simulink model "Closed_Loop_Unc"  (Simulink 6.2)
settings: Solver=ode23s  StartTime=0.0  StopTime=60  FixedStep=0.04  RelTol=1e-3
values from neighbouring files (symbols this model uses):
  Npv = 45    [run.m]
  r2d = 180/pi    (= 57.2957795131)    [run.m]    (also in Pl.m; pl.m; start.m)
undefined symbols (not defined in the file or in its folder): Ac, As, At, Au, Bc, Bs, Bt, Bu, Cc, Cs, Ct, Cu, Dc, Ds, Dt, Du

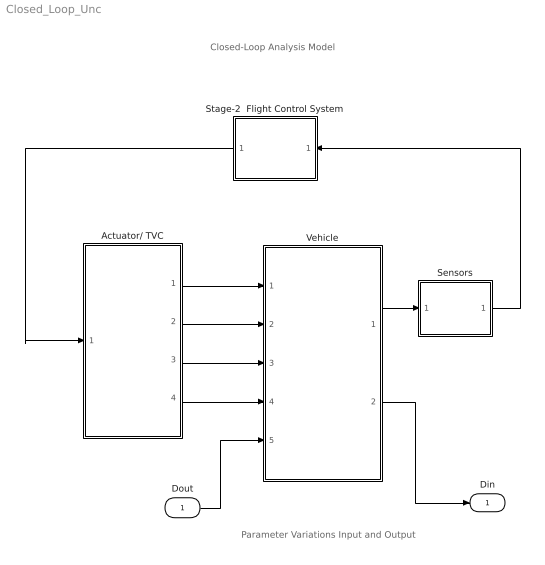
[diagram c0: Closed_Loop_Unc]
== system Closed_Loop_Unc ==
  note: Closed-Loop Analysis Model
  note: Parameter Variations Input and Output
  Dout : Inport  Port=1  LatchInput=off
  Actuator/ TVC : Subsystem
  Sensors : Subsystem
  Stage-2  Flight Control System : Subsystem  Orientation=left
  Vehicle : Subsystem
  Din : Outport
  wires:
  Vehicle/1(meas) -> Sensors/1(meas)
  Actuator/ TVC/1(DY) -> Vehicle/1(DY)
  Actuator/ TVC/2(DY-dd) -> Vehicle/2(DY_dd)
  Actuator/ TVC/3(DZ) -> Vehicle/3(DZ)
  Actuator/ TVC/4(DZ-dd) -> Vehicle/4(DZ_dd)
  Sensors/1(sens) -> Stage-2  Flight Control System/1(sens)
  Stage-2  Flight Control System/1(TVC) -> Actuator/ TVC/1(TVC)
  Vehicle/2(Din) -> Din/1
  Dout/1 -> Vehicle/5(Dout)

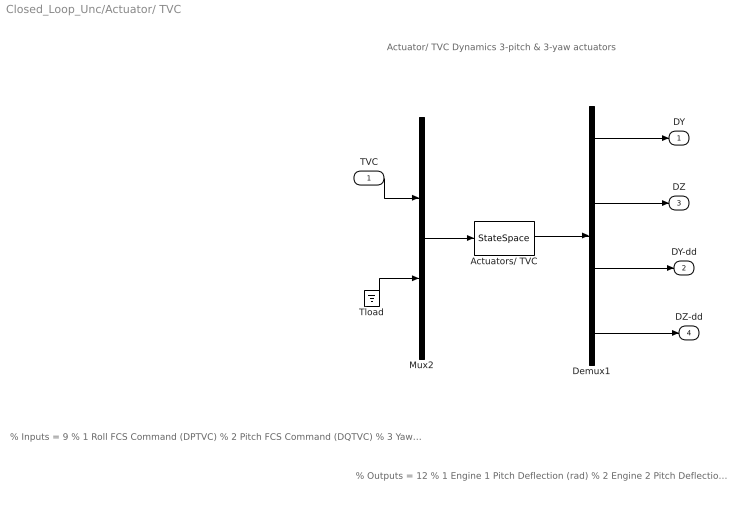
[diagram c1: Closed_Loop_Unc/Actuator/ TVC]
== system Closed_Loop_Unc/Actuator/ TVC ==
  note: % Outputs = 12 % 1 Engine 1 Pitch Deflection (rad) % 2 Engine 2 Pitch Deflection (rad) % 3 Engine 3 Pitch Deflection (rad) % 4 Engine 1 Yaw Deflection (rad) % 5 Engine 2 Yaw Deflection (rad) % 6 Engine 3 Yaw Deflection (rad) % 7 Engine 1 Pitch Accelerat (rad/sec^2) % 8 Engine 2 Pitch Accelerat (rad/sec^2) % 9 Engine 3 Pitch Accelerat (rad/sec^2) % 10 Engine 1 Yaw Accelerat (rad/sec^2) % 11 Engine 2 Yaw Accelerat (rad/sec^2) % 12 Engine 3 Yaw Accelerat (rad/sec^2)
  note: % Inputs = 9 % 1 Roll FCS Command (DPTVC) % 2 Pitch FCS Command (DQTVC) % 3 Yaw FCS Command (DRTVC) % 4 Engine 1 Pitch Load-Torque TLY1 % 5 Engine 2 Pitch Load-Torque TLY2 % 6 Engine 3 Pitch Load-Torque TLY3 % 7 Engine 1 Yaw Load-Torque TLZ1 % 8 Engine 2 Yaw Load-Torque TLZ2 % 9 Engine 3 Yaw Load-Torque TLZ3
  note: Actuator/ TVC Dynamics 3-pitch & 3-yaw actuators
  TVC : Inport  Port=1  LatchInput=off
  Actuators/ TVC : StateSpace  A=At  B=Bt  C=Ct  D=Dt
  Demux1 : Demux  Outputs=[3, 3, 3, 3]
  Mux2 : Mux  Inputs="[3,  6]"
  Tload : Ground
  DY : Outport
  DY-dd : Outport  Port=2
  DZ : Outport  Port=3
  DZ-dd : Outport  Port=4
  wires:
  Demux1/3 -> DY-dd/1
  Demux1/4 -> DZ-dd/1
  Demux1/2 -> DZ/1
  Demux1/1 -> DY/1
  TVC/1 -> Mux2/1
  Tload/1 -> Mux2/2
  Actuators/ TVC/1 -> Demux1/1
  Mux2/1 -> Actuators/ TVC/1

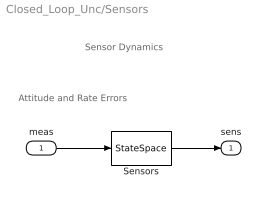
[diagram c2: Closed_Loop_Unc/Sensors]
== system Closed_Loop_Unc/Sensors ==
  note: Attitude and Rate Errors
  note: Sensor Dynamics
  meas : Inport  Port=1  LatchInput=off
  Sensors : StateSpace  A=As  B=Bs  C=Cs  D=Ds
  sens : Outport
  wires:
  Sensors/1 -> sens/1
  meas/1 -> Sensors/1

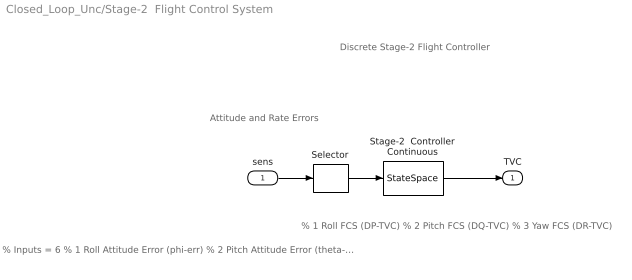
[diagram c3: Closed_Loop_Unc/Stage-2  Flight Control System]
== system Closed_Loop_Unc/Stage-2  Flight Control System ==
  note: Discrete Stage-2 Flight Controller
  note: Attitude and Rate Errors
  note: % Inputs = 6 % 1 Roll Attitude Error (phi-err) % 2 Pitch Attitude Error (theta-err) % 3 Yaw Attitude Error (psi-err) % 4 Roll Rate Error (p-err) % 5 Pitch Rate Error (q-err) % 6 Yaw Rate Error (r-err)
  note: % 1 Roll FCS (DP-TVC) % 2 Pitch FCS (DQ-TVC) % 3 Yaw FCS (DR-TVC)
  sens : Inport  Port=1  LatchInput=off
  Selector : Selector  Elements=[1 3 5 2 4 6]  InputPortWidth=6
  Stage-2  Controller Continuous : StateSpace  A=Ac  B=Bc  C=Cc  D=Dc
  TVC : Outport
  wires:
  sens/1 -> Selector/1
  Stage-2  Controller Continuous/1 -> TVC/1
  Selector/1 -> Stage-2  Controller Continuous/1

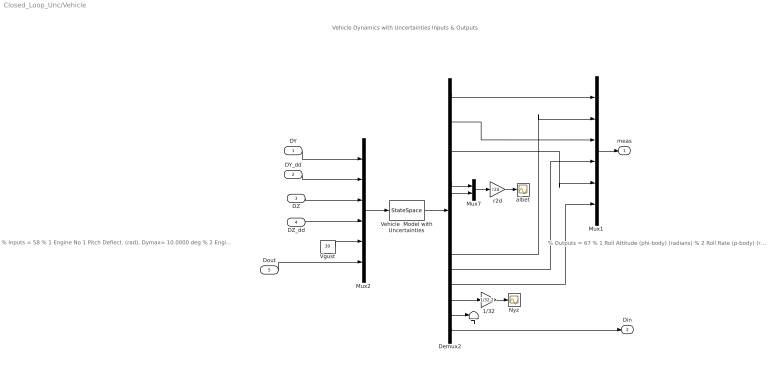
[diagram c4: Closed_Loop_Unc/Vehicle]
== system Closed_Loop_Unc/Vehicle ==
  note: Vehicle Dynamics with Uncertainties Inputs & Outputs
  note: % Outputs = 67 % 1 Roll Attitude (phi-body) (radians) % 2 Roll Rate (p-body) (rad/sec) % 3 Pitch Attitude (thet-bdy) (radians) % 4 Pitch Rate (q-body) (rad/sec) % 5 Yaw Attitude (psi-body) (radians) % 6 Yaw Rate (r-body) (rad/sec) % 7 Angle of attack, alfa, (radians) % 8 Angle of sideslip, beta, (radian) % 9 Change in Altitude, delta-h, (feet) % 10 Forward Acceleration (V-dot) (ft/sec) % 11 Cross Range Velocity (Vcr) (ft/sec) % 12 Rate-Gyro # 1, Roll Rate (Body) (rad/sec) % 13 Rate-Gyro # 2, Pitch Rate (Body) (rad/sec) % 14 Rate-Gyro # 3, Yaw Rate (Body) (rad/sec) % 15 Accelerom # 1, (along Z), (ft/sec^2) Translat. Acceler % 16 Accelerom # 2, (along Y), (ft/sec^2) Translat. Acceler % 17 Ptch Load-Torque Tly for Engine: 1,(ft-lb) % 18 Ptch Load-Torque Tly for Engine: 2,(ft-lb) % 19 Ptch Load-Torque Tly for Engine: 3,(ft-lb) % 20 Yaw Load-Torque Tlz for Engine: 1,(ft-lb) % 21 Yaw Load-Torque Tlz for Engine: 2,(ft-lb) % 22 Yaw Load-Torque Tlz for Engine: 3,(ft-lb) Variations % 23 Cl_beta : -44.321 % Variation % 24 Cm_alpha : -13.472 % Variation % 25 Cn_beta : 23.053 % Variation % 26 Ca_alpha : 31.831 % Variation % 27 Cz_alpha : -6.829 % Variation % 28 Cy_beta : -25.185 % Variation % 29 Cm_0 : 35.804 % Variation % 30 CZ_0 : 230.769 % Variation % 31 CA_0 : 13.937 % Variation % 32 I_xx : 6.615 % Variation % 33 I_yy : 3.435 % Variation % 34 I_zz : 3.616 % Variation % 35 Xcg locat: -1.050 % Variation % 36 Xcg locat: -1.050 % Variation % 37 Thr_eng 1: 2.046 % Variation % 38 Thr_eng 1: 2.046 % Variation % 39 Thr_eng 2: 2.046 % Variation % 40 Thr_eng 2: 2.046 % Variation % 41 Thr_eng 3: 2.046 % Variation % 42 Thr_eng 3: 2.046 % Variation % 43 M_slosh 1: 1.660 % Variation % 44 M_slosh 1: 1.660 % Variation % 45 X_slosh 1: -3.093 % Variation % 46 X_slosh 1: -3.093 % Variation % 47 Z_slosh 1: -1.500 % Variation % 48 Z_slosh 1: -1.500 % Variation % 49 Wslsh_Y 1: 2.257 % Variation % 50 Wslsh_Z 1: 2.257 % Variation % 51 M_slosh 2: 10.762 % Variation % 52 M_slosh 2: 10.762 % Variation
  note: % Inputs = 58 % 1 Engine No 1 Pitch Deflect. (rad), Dymax= 10.0000 deg % 2 Engine No 2 Pitch Deflect. (rad), Dymax= 10.0000 deg % 3 Engine No 3 Pitch Deflect. (rad), Dymax= 10.0000 deg % 4 Engine No 1 Pitch Acceleration (rad/sec^2) % 5 Engine No 2 Pitch Acceleration (rad/sec^2) % 6 Engine No 3 Pitch Acceleration (rad/sec^2) % 7 Engine No 1 Yaw Deflect. (rad), Dzmax= 10.0000 deg % 8 Engine No 2 Yaw Deflect. (rad), Dzmax= 10.0000 deg % 9 Engine No 3 Yaw Deflect. (rad), Dzmax= 10.0000 deg % 10 Engine No 1 Yaw Acceleration (rad/sec^2) % 11 Engine No 2 Yaw Acceleration (rad/sec^2) % 12 Engine No 3 Yaw Acceleration (rad/sec^2) % 13 Wind Gust Azim, Elev Angles=( 45.0 90.0) (deg) Variations = 45 % 14 Cl_beta : -44.321 % Variation % 15 Cm_alpha : -13.472 % Variation % 16 Cn_beta : 23.053 % Variation % 17 Ca_alpha : 31.831 % Variation % 18 Cz_alpha : -6.829 % Variation % 19 Cy_beta : -25.185 % Variation % 20 Cm_0 : 35.804 % Variation % 21 CZ_0 : 230.769 % Variation % 22 CA_0 : 13.937 % Variation % 23 I_xx : 6.615 % Variation % 24 I_yy : 3.435 % Variation % 25 I_zz : 3.616 % Variation % 26 Xcg locat: -1.050 % Variation % 27 Xcg locat: -1.050 % Variation % 28 Thr_eng 1: 2.046 % Variation % 29 Thr_eng 1: 2.046 % Variation % 30 Thr_eng 2: 2.046 % Variation % 31 Thr_eng 2: 2.046 % Variation % 32 Thr_eng 3: 2.046 % Variation % 33 Thr_eng 3: 2.046 % Variation % 34 M_slosh 1: 1.660 % Variation % 35 M_slosh 1: 1.660 % Variation % 36 X_slosh 1: -3.093 % Variation % 37 X_slosh 1: -3.093 % Variation % 38 Z_slosh 1: -1.500 % Variation % 39 Z_slosh 1: -1.500 % Variation % 40 Wslsh_Y 1: 2.257 % Variation % 41 Wslsh_Z 1: 2.257 % Variation % 42 M_slosh 2: 10.762 % Variation % 43 M_slosh 2: 10.762 % Variation % 44 M_slosh 2: 10.762 % Variation % 45 X_slosh 2: -1.596 % Variation % 46 X_slosh 2: -1.596 % Variation % 47 X_slosh 2: -1.596 % Variation % 48 Z_slosh 2: -1.500 % Variation % 49 Z_slosh 2: -1.500 % Variation % 50 Z_slosh 2: -1.500 % Variation % 51 Wslsh_Y 2: 2.379 % Variation % 52 Wslsh
  DY : Inport  Port=1  LatchInput=off
  DY_dd : Inport  Port=2  LatchInput=off
  DZ : Inport  Port=3  LatchInput=off
  DZ_dd : Inport  Port=4  PortDimensions=3  LatchInput=off
  Dout : Inport  Port=5  PortDimensions=Npv  LatchInput=off
  1/32 : Gain  Gain=1/32.2
  Demux2 : Demux  Outputs=[1, 1, 1, 1, 1, 1, 1, 1, 1, 1, 1, 1, 1, 1, 2, 6, Npv]
  Mux1 : Mux  Inputs=6
  Mux2 : Mux  Inputs=[3, 3, 3, 3, 1, Npv]
  Mux7 : Mux  Inputs=2
  Nyz : Scope
  TL : Terminator
  Vehicle  Model with Uncertainties : StateSpace  A=Au  B=Bu  C=Cu  D=Du
  Vgust : Constant  Value=30
  albet : Scope
  r2d : Gain  Gain=r2d
  meas : Outport
  Din : Outport  Port=2
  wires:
  Mux1/1 -> meas/1
  Demux2/5 -> Mux1/5
  Demux2/3 -> Mux1/3
  Demux2/1 -> Mux1/1
  Demux2/8 -> Mux7/2
  Demux2/7 -> Mux7/1
  Demux2/12 -> Mux1/2
  Demux2/13 -> Mux1/4
  Demux2/14 -> Mux1/6
  Mux2/1 -> Vehicle  Model with Uncertainties/1
  r2d/1 -> albet/1
  Mux7/1 -> r2d/1
  1/32/1 -> Nyz/1
  Demux2/15 -> 1/32/1
  Demux2/16 -> TL/1
  Vehicle  Model with Uncertainties/1 -> Demux2/1
  Dout/1 -> Mux2/6
  Demux2/17 -> Din/1
  Vgust/1 -> Mux2/5
  DZ_dd/1 -> Mux2/4
  DZ/1 -> Mux2/3
  DY_dd/1 -> Mux2/2
  DY/1 -> Mux2/1
